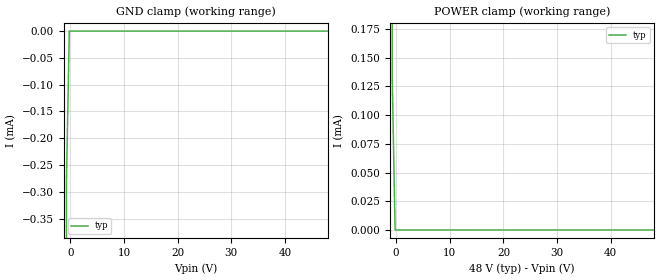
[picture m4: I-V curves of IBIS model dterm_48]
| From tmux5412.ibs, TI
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| dterm_48
[Model]   dterm_48
Model_type   Terminator
|   typ   min   max
C_comp   1.008417e-11   NA   NA
[Voltage Range]   48   NA   NA
[Temperature Range]   27   NA   NA
[Power Clamp Reference]   48   NA   NA
[GND Clamp Reference]   0   NA   NA
[GND Clamp]
|   Voltage   I(typ)   I(min)   I(max)
-5V       -2.839A    NA         NA
-1.253V   -90.92mA   NA         NA
-717.2mV  -285.5uA   NA         NA
-181.8mV  -1.964nA   NA         NA
48V       4.289nA    NA         NA
[POWER Clamp]
|   Voltage   I(typ)   I(min)   I(max)
-5V       2.611A     NA         NA
-1.252V   80.72mA    NA         NA
-717.2mV  133.1uA    NA         NA
-181.8mV  4.329nA    NA         NA
48V       -1.892nA   NA         NA
